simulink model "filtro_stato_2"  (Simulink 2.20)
settings: Solver=VariableStepDiscrete  StartTime=0.0  StopTime=50.0  RelTol=1e-3  AbsTol=1e-6
undefined symbols (not defined in the file or in its folder): k1, k2, T
libraries: simulink x2

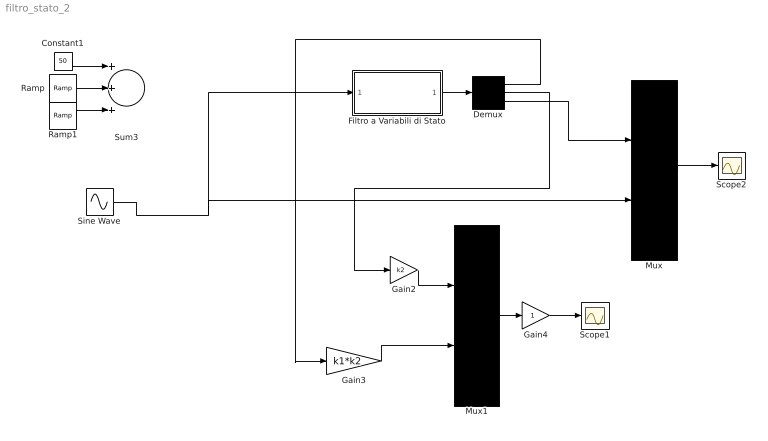
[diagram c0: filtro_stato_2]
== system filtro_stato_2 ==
  Constant1 : Constant  Value=50
  Demux : Demux  Outputs=3
  Filtro a Variabili di Stato : Subsystem  mask{T=T, k1=5, k2=10}
      mask prompts: T "Sample Time"; k1 "Gudagno k1"; k2 "Guadagno k2"
      mask init:
      | A=[0,-1,-1;k1*T,1,0;0,k2*T,1]
  Gain2 : Gain  Gain=k2
  Gain3 : Gain  Gain=k1*k2
  Gain4 : Gain  Gain=1
  Mux : Mux  Inputs=2
  Mux1 : Mux  Inputs=2
  Ramp : simulink/Sources/Ramp  slope=-50  start=10  X0=0
  Ramp1 : simulink/Sources/Ramp  slope=+100  start=20  X0=0
  Scope1 : Scope
  Scope2 : Scope
  Sine Wave : Sin  Amplitude=50  Frequency=.5  Phase=0  SampleTime=0
  Sum3 : Sum  Inputs=+++
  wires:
  Constant1/1 -> Sum3/1
  Ramp/1 -> Sum3/2
  Ramp1/1 -> Sum3/3
  Gain2/1 -> Mux1/1
  Gain3/1 -> Mux1/2
  Mux1/1 -> Gain4/1
  Gain4/1 -> Scope1/1
  Mux/1 -> Scope2/1
  Demux/3 -> Mux/1
  Demux/2 -> Gain2/1
  Demux/1 -> Gain3/1
  Filtro a Variabili di Stato/1(Out1) -> Demux/1
  Sine Wave/1 -> Mux/2, Filtro a Variabili di Stato/1(In1)

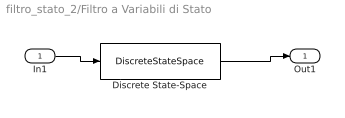
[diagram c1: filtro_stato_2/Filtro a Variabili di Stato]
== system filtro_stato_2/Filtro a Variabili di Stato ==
  In1 : Inport  Port=1  PortWidth=-1  SampleTime=-1
  Discrete State-Space : DiscreteStateSpace  A=A  B=[1;0;0]  C=[1,0,0;0,1,0;0,0,1]  D=[0;0;0]  X0=0  SampleTime=0.01
  Out1 : Outport  Port=1
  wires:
  In1/1 -> Discrete State-Space/1
  Discrete State-Space/1 -> Out1/1
